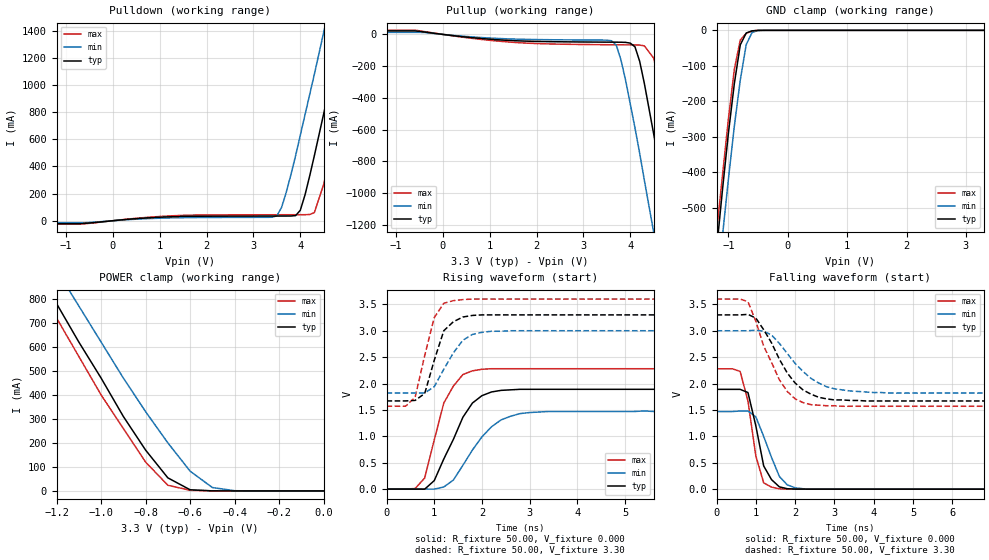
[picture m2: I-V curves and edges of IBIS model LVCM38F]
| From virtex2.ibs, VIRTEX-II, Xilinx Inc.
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|   Model LVCM38F
[Model]   LVCM38F
Model_type   I/O
Polarity   Non-Inverting
Enable   Active-Low
Vinh = 2.0V
Vinl = 0.8V
Vmeas =   1.65V
Cref =  35.00pF
Rref =   1.00M
Vref =  0.000V
C_comp   7.00pF   6.00pF   8.00pF
[Temperature Range]   25.00   100.00   0.000
[Voltage Range]   3.30V   3.00V   3.60V
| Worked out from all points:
|   slope of the pulldown table from 0 to 0.495 V, typ, clamps not added: 32.6 ohm
|   slope of the pullup table from 0 to 0.495 V, typ, clamps not added: 29.6 ohm
|   GND clamp passes 1 mA (typ) near -0.57 V on its own axis
|   POWER clamp passes 1 mA (typ) near -0.52 V on its own axis
|   rising waveform, R_fixture 50.00, V_fixture 0.000: 20-80 % time 606ps typ, 707ps min, 453ps max; typ from 0 V to 1.89 V
|   rising waveform, R_fixture 50.00, V_fixture 3.30: 20-80 % time 332ps typ, 483ps min, 325ps max; typ from 1.67 V to 3.3 V
|   falling waveform, R_fixture 50.00, V_fixture 0.000: 20-80 % time 347ps typ, 465ps min, 323ps max; typ from 1.89 V to 0 V
|   falling waveform, R_fixture 50.00, V_fixture 3.30: 20-80 % time 785ps typ, 903ps min, 693ps max; typ from 3.3 V to 1.67 V
[Pulldown]
| voltage   I(typ)   I(min)   I(max)
-3.3V     -21.47mA   -14.42mA   -24.67mA
-700mV    -21.47mA   -14.42mA   -24.67mA
1.3V      29.85mA    21.41mA    36.81mA
3.5V      34.44mA    36.13mA    44.01mA
3.7V      34.53mA    210mA      44.1mA
4V        77.1mA     630mA      44.22mA
4.3V      480mA      1.08A      60mA
4.5V      790mA      1.39A      270mA
4.9V      1.44A      2.02A      900mA
5.1V      1.77A      2.33A      1.22A
5.3V      2.1A       2.65A      1.55A
6.6V      4.26A      4.71A      3.71A
[Pullup]
| voltage   I(typ)   I(min)   I(max)
-3.3V     21.9mA     12.73mA    26.65mA
-600mV    21.9mA     12.73mA    26.65mA
3.6V      -48.95mA   -40.18mA   -65.29mA
3.8V      -49.31mA   -160mA     -65.71mA
4.1V      -78.6mA    -590mA     -66.32mA
4.3V      -310mA     -920mA     -72.41mA
4.5V      -630mA     -1.25A     -150mA
4.7V      -970mA     -1.58A     -430mA
4.9V      -1.32A     -1.92A     -760mA
5.1V      -1.66A     -2.26A     -1.1A
5.3V      -2.01A     -2.6A      -1.45A
6.6V      -4.32A     -4.84A     -3.74A
[GND_clamp]
| voltage   I(typ)   I(min)   I(max)
-3.3V     -4.3A      -4.31A     -4.26A
-1.2V     -620mA     -740mA     -570mA
-1.1V     -450mA     -580mA     -410mA
-1V       -290mA     -420mA     -250mA
-900mV    -150mA     -270mA     -110mA
-800mV    -41.03mA   -140mA     -27.28mA
-700mV    -7.6mA     -40.21mA   -8.18mA
-600mV    -1.42mA    -5.61mA    -1.62mA
-500mV    -130uA     -670uA     -130uA
3.3V      67.85pA    43.48uA    45.6pA
[POWER_clamp]
| voltage   I(typ)   I(min)   I(max)
-3.3V     4.25A      4.22A      4.2A
-1.3V     940mA      1.07A      880mA
-1.2V     780mA      920mA      720mA
-1.1V     620mA      770mA      560mA
-1V       470mA      620mA      400mA
-900mV    310mA      470mA      260mA
-800mV    170mA      330mA      120mA
-700mV    54.34mA    200mA      23.62mA
-600mV    4.76mA     82.21mA    2.52mA
-500mV    280uA      14.02mA    260uA
-400mV    16.9uA     860uA      14.85uA
0V        67.85pA    2.04nA     61.89pA
[Ramp]
| variable   typ   min   max
dV/dt_r   1.14/0.53n   0.88/0.70n   1.37/0.41n
dV/dt_f   0.98/0.74n   0.71/0.90n   1.22/0.62n
R_load = 50.00
[Rising Waveform]
R_fixture = 50.00
V_fixture = 0.000
| time   V(typ)   V(min)   V(max)
0s        0V         0V         0V
600ps     -1.1mV     45.89uV    10.08mV
800ps     -2.02mV    -450uV     210mV
1ns       160mV      -870uV     930mV
1.2ns     570mV      39.42mV    1.63V
1.6ns     1.36V      450mV      2.17V
1.8ns     1.63V      740mV      2.24V
2.4ns     1.87V      1.31V      2.28V
3ns       1.89V      1.45V      2.28V
10ns      1.89V      1.47V      2.28V
[Rising Waveform]
R_fixture = 50.00
V_fixture = 3.30
V_fixture_min = 3.00
V_fixture_max = 3.60
| time   V(typ)   V(min)   V(max)
0s        1.67V      1.82V      1.57V
400ps     1.67V      1.82V      1.57V
600ps     1.68V      1.82V      1.74V
800ps     1.81V      1.82V      2.53V
1ns       2.44V      1.94V      3.25V
1.2ns     3V         2.27V      3.52V
1.4ns     3.17V      2.58V      3.57V
1.8ns     3.29V      2.93V      3.6V
2.2ns     3.3V       2.99V      3.6V
10ns      3.3V       3V         3.6V
[Falling Waveform]
R_fixture = 50.00
V_fixture = 0.000
| time   V(typ)   V(min)   V(max)
0s        1.89V      1.47V      2.28V
600ps     1.89V      1.48V      2.23V
800ps     1.83V      1.48V      1.67V
1ns       1.2V       1.37V      630mV
1.2ns     440mV      1V         120mV
1.4ns     180mV      600mV      37.98mV
1.6ns     43.13mV    240mV      6.87mV
1.8ns     8.57mV     81.66mV    1.29mV
2.2ns     800uV      8.03mV     240uV
10ns      4.36uV     3.55uV     1.59uV
[Falling Waveform]
R_fixture = 50.00
V_fixture = 3.30
V_fixture_min = 3.00
V_fixture_max = 3.60
| time   V(typ)   V(min)   V(max)
0s        3.3V       3V         3.6V
800ps     3.31V      3V         3.55V
1ns       3.24V      3.01V      3.18V
1.2ns     3.02V      2.99V      2.71V
1.6ns     2.46V      2.76V      2.07V
1.8ns     2.2V       2.57V      1.85V
2.2ns     1.88V      2.23V      1.64V
2.8ns     1.71V      1.94V      1.58V
3.4ns     1.68V      1.86V      1.57V
10ns      1.67V      1.82V      1.57V
